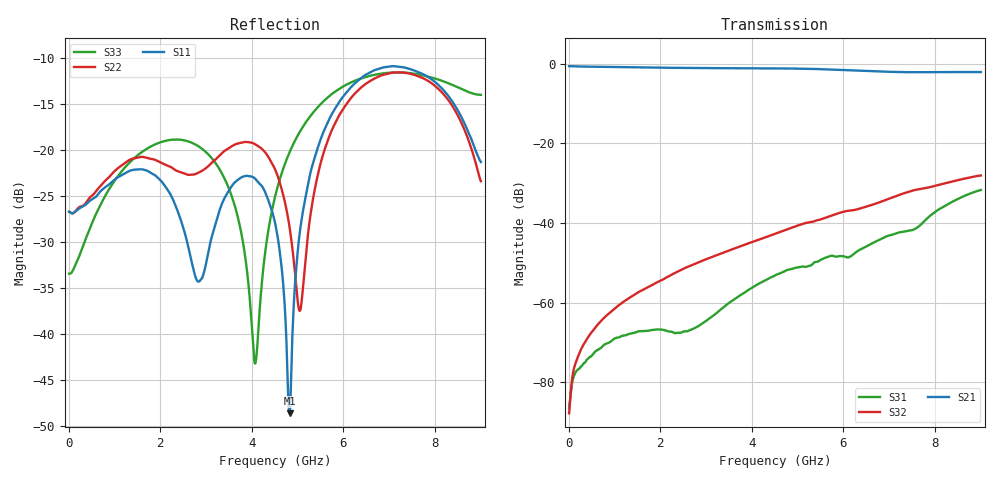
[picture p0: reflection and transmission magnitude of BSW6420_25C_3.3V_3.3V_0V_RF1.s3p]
!Agilent Technologies,N5230C,MY49001333,A.09.33.09
!Agilent N5230C: A.09.33.09
!Date: Monday, September 23, 2024 13:22:16
!Correction: S11(Full 3 Port(1,2,3))
!S12(Full 3 Port(1,2,3))
!S13(Full 3 Port(1,2,3))
!S21(Full 3 Port(1,2,3))
!S22(Full 3 Port(1,2,3))
!S23(Full 3 Port(1,2,3))
!S31(Full 3 Port(1,2,3))
!S32(Full 3 Port(1,2,3))
!S33(Full 3 Port(1,2,3))
!S3P File: Measurements: <S11,S12,S13>,
!<S21,S22,S23>,
!<S31,S32,S33>:
# Hz S  MA  R 50
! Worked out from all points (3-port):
!   901 points, 10 MHz to 9.01 GHz, reference 50 ohm
!   strongest paths, dB at 10 MHz, 2.26 GHz, 4.51 GHz, 6.76 GHz, 9.01 GHz:
!     S21: -0.6, -1.0, -1.2, -1.9, -2.1
!     S32: -87.8, -52.9, -42.7, -34.9, -28.1
!     S31: -86.4, -67.4, -53.2, -44.4, -31.7
!   lowest |S11| = -48.6 dB at 4.83 GHz (marker M1), VSWR 1.01, Z = 49.7 - j0.216 ohm
!   |S11| at or under -10 dB: start of sweep to end of sweep
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1e7  0.04627 -4.3  0.931 -2.4  4.311e-05 -3.0
     0.931 -2.3  0.04622 -4.1  4.338e-05 25.1
     4.801e-05 -11.7  4.073e-05 -7.4  0.0213 -7.1
1.67e9  0.07786 117.8  0.8965 -170.6  0.0004446 -117.8
        0.8956 -170.7  0.09131 146.8  0.001516 -45.2
        0.0004406 -118.1  0.001502 -45.1  0.1003 149.5
2.74e9  0.02187 49.3  0.884 80.9  0.0004676 75.2
        0.8839 80.8  0.07368 88.0  0.003088 -132.2
        0.000474 75.3  0.003038 -131.7  0.1082 66.0
4.08e9  0.06976 27.1  0.8719 -54.9  0.001625 -124.7
        0.8731 -55.2  0.1074 9.5  0.006089 107.7
        0.001619 -124.5  0.005963 107.7  0.006922 -120.8
4.51e9  0.04035 -13.7  0.8717 -98.7  0.002195 -177.0
        0.8723 -98.9  0.07868 -32.9  0.007387 68.2
        0.002195 -177.0  0.007301 68.1  0.0556 126.1
4.83e9  0.003709 -144.1  0.8697 -131.5  0.002595 143.6
        0.87 -131.6  0.03784 -74.6  0.008617 38.1
        0.00261 144.4  0.008533 38.0  0.0975 99.6
6.06e9  0.2039 10.3  0.8349 102.1  0.003837 15.7
        0.8298 102.3  0.176 8.9  0.01417 -82.0
        0.003731 16.8  0.01408 -82.4  0.226 2.7
7.07e9  0.2856 -94.7  0.7997 -0.7  0.007337 -76.5
        0.7891 -0.2  0.2634 -88.2  0.0204 -179.0
        0.007123 -77.8  0.02087 178.9  0.2639 -82.7
8e9  0.2355 165.4  0.7928 -95.8  0.01352 -157.7
     0.783 -95.3  0.2241 -173.4  0.02734 83.2
     0.01362 -159.5  0.02916 81.7  0.2453 -171.3
9.01e9  0.08615 34.3  0.7897 158.7  0.02543 84.7
        0.7848 158.6  0.06779 92.4  0.03715 -23.6
        0.02597 83.8  0.03947 -22.6  0.1997 65.4
